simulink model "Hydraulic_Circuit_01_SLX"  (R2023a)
settings: Solver=ode23s  StartTime=0.0  StopTime=10.0  MaxStep=0.001  RelTol=1e-3
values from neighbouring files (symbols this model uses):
  C_4 = 0.001*m^3/Pa    (= 0.001)    [Hydraulic_Circuit_01_EQN.m]    (also in Hydraulic_Circuit_01_SLX_m.m; Electric_Circuit_01_EQN.m; Electric_Circuit_01_SLX_m.m; Electric_Circuit_06_EQN.m)
  C_6 = 0.001*m^3/Pa    (= 0.001)    [Hydraulic_Circuit_01_EQN.m]    (also in Hydraulic_Circuit_01_SLX_m.m; Electric_Circuit_01_EQN.m; Electric_Circuit_01_SLX_m.m; Electric_Circuit_03_EQN.m)
  L_3 = 10*Pa*sec^2/m^3    (= 10)    [Hydraulic_Circuit_01_EQN.m]    (also in Hydraulic_Circuit_01_SLX_m.m; Electric_Circuit_08_EQN.m = 0.002; Electric_Circuit_08_SLX_m.m = 0.002; Electric_Circuit_10_EQN.m = 0.002)
  L_5 = 10*Pa*sec^2/m^3    (= 10)    [Hydraulic_Circuit_01_EQN.m]    (also in Hydraulic_Circuit_01_SLX_m.m; BIG_EC_Simscape_EQN.m = 0.002; BIG_EC_Simscape_SLX_m.m = 0.002; Electric_Circuit_01_EQN.m = 0.002)
  P_1_0 = 10*Pa    (= 10)    [Hydraulic_Circuit_01_SLX_m.m]    (also in Hydraulic_Circuit_02_SLX_m.m; Hydraulic_Circuit_03_SLX_m.m; Hydraulic_Clutch_System_SLX_m.m)
  P_4_0 = 0*Pa    (= 0)    [Hydraulic_Circuit_01_SLX_m.m]
  P_6_0 = 0*Pa    (= 0)    [Hydraulic_Circuit_01_SLX_m.m]
  Q_3_0 = 0*m^3/sec    (= 0)    [Hydraulic_Circuit_01_SLX_m.m]
  Q_5_0 = 0*m^3/sec    (= 0)    [Hydraulic_Circuit_01_SLX_m.m]
  Q_8_0 = 0*m^3/sec    (= 0)    [Hydraulic_Circuit_01_SLX_m.m]
  R_2 = 10000*Pa/(m^3/sec)    (= 10000)    [Hydraulic_Circuit_01_EQN.m]    (also in Hydraulic_Circuit_01_SLX_m.m; BIG_EC_Simscape_EQN.m = 100; BIG_EC_Simscape_SLX_m.m = 100; Electric_Circuit_07_EQN.m = 100)
  R_7 = 10000*Pa/(m^3/sec)    (= 10000)    [Hydraulic_Circuit_01_EQN.m]    (also in Hydraulic_Circuit_01_SLX_m.m; BIG_EC_Simscape_EQN.m = 100; BIG_EC_Simscape_SLX_m.m = 100; Electric_Circuit_03_EQN.m = 100)
  Ts = Tfin/Nr_Ts_Points    (= 0.060003)    [Hydraulic_Circuit_01_SLX_m.m]    (also in BIG_EC_Simscape_SLX_m.m = 0.0003; Car_Dumper_SLX_m.m = 0.0022779; Electric_Circuit_01_SLX_m.m = 0.005; Electric_Circuit_02_SLX_m.m = 0.000480145)

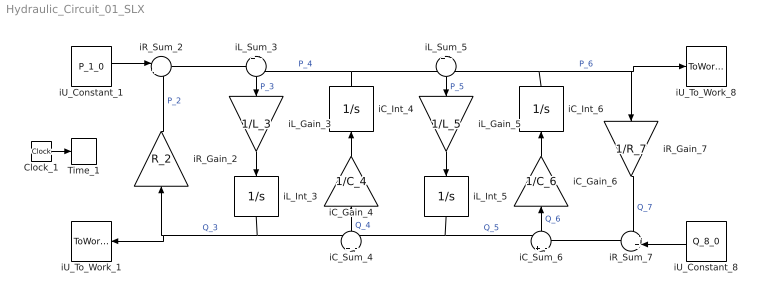
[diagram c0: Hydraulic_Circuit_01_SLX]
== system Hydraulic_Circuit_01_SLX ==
  Clock_1 : Clock
  Time_1 : ToWorkspace  VariableName=t  SaveFormat=Timeseries  SampleTime=Ts
  iC_Gain_4 : Gain  Gain=1/C_4  Multiplication=Matrix(K*u)
  iC_Gain_6 : Gain  Gain=1/C_6  Multiplication=Matrix(K*u)
  iC_Int_4 : Integrator  InitialCondition=P_4_0
  iC_Int_6 : Integrator  InitialCondition=P_6_0
  iC_Sum_4 : Sum  Inputs=+|-
  iC_Sum_6 : Sum  Inputs=+|-
  iL_Gain_3 : Gain  Gain=1/L_3  Multiplication=Matrix(K*u)
  iL_Gain_5 : Gain  Gain=1/L_5  Multiplication=Matrix(K*u)
  iL_Int_3 : Integrator  InitialCondition=Q_3_0
  iL_Int_5 : Integrator  InitialCondition=Q_5_0
  iL_Sum_3 : Sum  Inputs=+|-
  iL_Sum_5 : Sum  Inputs=+|-
  iR_Gain_2 : Gain  Gain=R_2  Multiplication=Matrix(K*u)
  iR_Gain_7 : Gain  Gain=1/R_7  Multiplication=Matrix(K*u)
  iR_Sum_2 : Sum  Inputs=|+-
  iR_Sum_7 : Sum  Inputs=++|
  iU_Constant_1 : Constant  Value=P_1_0
  iU_Constant_8 : Constant  Value=Q_8_0
  iU_To_Work_1 : ToWorkspace  VariableName=Q_1_0  SaveFormat=Timeseries  SampleTime=Ts
  iU_To_Work_8 : ToWorkspace  VariableName=P_8_0  SaveFormat=Timeseries  SampleTime=Ts
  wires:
  iU_Constant_1/1 -> iR_Sum_2/1
  iR_Sum_2/1 -> iL_Sum_3/1
  iL_Int_3/1 -> iU_To_Work_1/1, iR_Gain_2/1, iC_Sum_4/1  "Q_3"
  iR_Gain_2/1 -> iR_Sum_2/2  "P_2"
  iC_Int_4/1 -> iL_Sum_3/2, iL_Sum_5/1  "P_4"
  iL_Sum_3/1 -> iL_Gain_3/1  "P_3"
  iL_Gain_3/1 -> iL_Int_3/1
  iL_Int_5/1 -> iC_Sum_4/2, iC_Sum_6/1  "Q_5"
  iC_Sum_4/1 -> iC_Gain_4/1  "Q_4"
  iC_Gain_4/1 -> iC_Int_4/1
  iC_Int_6/1 -> iL_Sum_5/2, iU_To_Work_8/1, iR_Gain_7/1  "P_6"
  iL_Sum_5/1 -> iL_Gain_5/1  "P_5"
  iL_Gain_5/1 -> iL_Int_5/1
  iR_Sum_7/1 -> iC_Sum_6/2
  iC_Sum_6/1 -> iC_Gain_6/1  "Q_6"
  iC_Gain_6/1 -> iC_Int_6/1
  iU_Constant_8/1 -> iR_Sum_7/2
  iR_Gain_7/1 -> iR_Sum_7/1  "Q_7"
  Clock_1/1 -> Time_1/1
